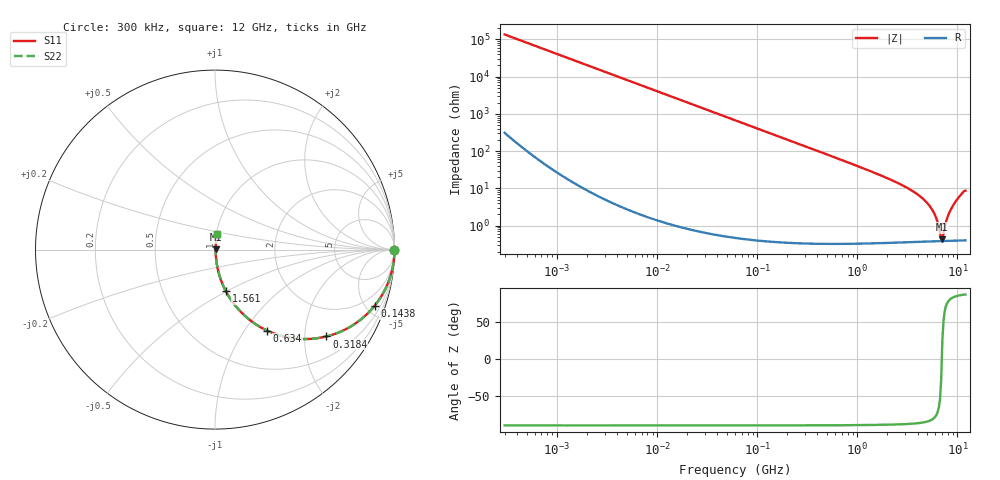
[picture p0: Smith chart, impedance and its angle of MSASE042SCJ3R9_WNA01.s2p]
! MSASE042SCJ3R9_WNA01  S-PARAMETER MODEL  ( General Type )
! Model Generated by TAIYO YUDEN Corporation (http://www.ty-top.com)
! Version 1.0
! TAIYO YUDEN Control No. 120810
! Copyright(c) 2012 TAIYO YUDEN CO.,LTD. All Rights Reserved.
! Product Description (link to TY-COMPAS)
! https://ds.yuden.co.jp/TYCOMPAS/or/detail?pn=MSASE042SCJ3R9BWNA01&u=M
! Products Name : Multilayer Ceramic Capacitors
! Characteristics :
!  Capacitance : 3.9 pF , Rated Voltage : 16V , TCC : CJ / C0J
!  Case Size : 0.4 x 0.2 / 0.016 x 0.008 [mm/inch] , Thickness : 0.2 / 0.008 [mm/inch]
!  (Conditions: Temperature = 25 degC , DC Bias Current/Voltage = 0A / 0V)
! External Node Assignments :
!  1  o---| |---o  2
! GND o---------o GND
! Frequency Range : 0.3MHz  -  12000MHz  [ 401 STEP ]
# MHz S RI R 50
! Freq[MHz].  S11 Real  S11 Imag  S21 Real  S21 Imag  S12 Real  S12 Imag  S22 Real  S22 Imag
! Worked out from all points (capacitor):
!   401 points, 300 kHz to 12 GHz, reference 50 ohm
!   read as one part in series: C = 3.9 pF near 316.3 kHz
!   lowest |Z| = 427 mohm at 7.064 GHz (marker M1)
!   series resonance near 6.977 GHz, so ESL is about 130 pH
!   S11 on the Smith chart (normalised r, x): 300 kHz: open; 143.8 MHz: 1.01, -5.68; 318.4 MHz: 1.01, -2.56; 634 MHz: 1.01, -1.28; 1.561 GHz: 1.01, -0.50; 12 GHz: 1.01, +0.17
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0.3  1 -0.000735  2.22e-06 0.000735  2.22e-06 0.000735  1 -0.000735
1.769972  1 -0.00433  2.08e-05 0.00433  2.08e-05 0.00433  1 -0.00433
10.44266  0.9993 -0.0256  0.000662 0.0256  0.000662 0.0256  0.9993 -0.0256
60  0.9788 -0.1438  0.0212 0.1438  0.0212 0.1438  0.9788 -0.1438
143.8206  0.8893 -0.3132  0.1107 0.3132  0.1107 0.3132  0.8893 -0.3132
318.4019  0.6207 -0.4839  0.3793 0.4839  0.3793 0.4839  0.6207 -0.4839
353.9943  0.5696 -0.4937  0.4304 0.4937  0.4304 0.4937  0.5696 -0.4937
634.0297  0.2908 -0.4516  0.7092 0.4516  0.7092 0.4516  0.2908 -0.4516
968.706  0.148 -0.3512  0.852 0.3512  0.852 0.3512  0.148 -0.3512
1560.575  0.0611 -0.2328  0.9389 0.2328  0.9389 0.2328  0.0611 -0.2328
2088.533  0.0339 -0.1715  0.9661 0.1715  0.9661 0.1715  0.0339 -0.1715
3547.679  0.0108 -0.0844  0.9892 0.0844  0.9892 0.0844  0.0108 -0.0844
4875.354  0.00557 -0.0428  0.9944 0.0428  0.9944 0.0428  0.00557 -0.0428
5868.704  0.00422 -0.0206  0.9958 0.0206  0.9958 0.0206  0.00422 -0.0206
6188.031  0.00402 -0.0144  0.996 0.0144  0.996 0.0144  0.00402 -0.0144
6699.894  0.00387 -0.00522  0.9961 0.00522  0.9961 0.00522  0.00387 -0.00522
7064.448  0.00386 0.00179  0.9961 -0.00179  0.9961 -0.00179  0.00386 0.00179
7254.098  0.00389 0.00487  0.9961 -0.00487  0.9961 -0.00487  0.00389 0.00487
8064.993  0.00423 0.0181  0.9958 -0.0181  0.9958 -0.0181  0.00423 0.0181
8732.115  0.00477 0.0291  0.9952 -0.0291  0.9952 -0.0291  0.00477 0.0291
10511.28  0.00771 0.0609  0.9923 -0.0609  0.9923 -0.0609  0.00771 0.0609
12000  0.0114 0.0855  0.9886 -0.0855  0.9886 -0.0855  0.0114 0.0855
